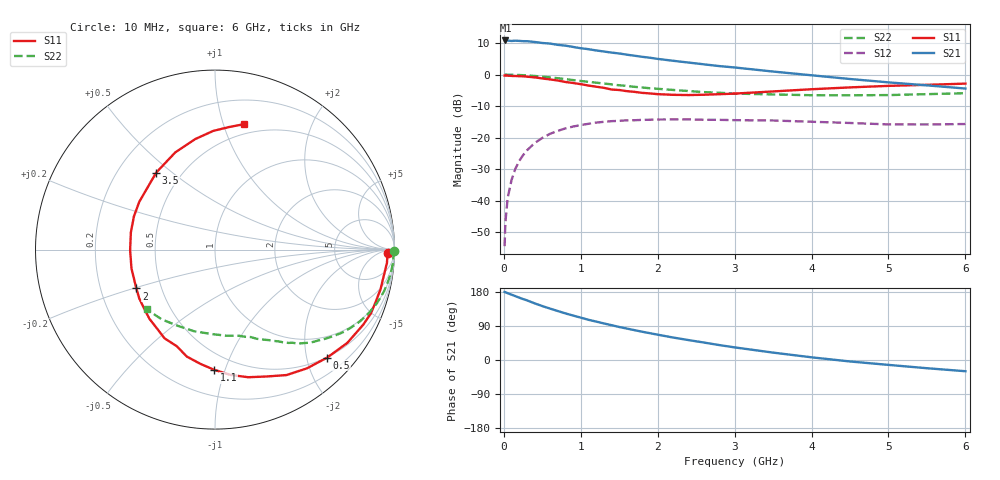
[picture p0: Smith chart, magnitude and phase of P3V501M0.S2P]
! SIEMENS Small Signal Semiconductors
! BFP181
! Si NPN RF Bipolar Junction Transistor in SOT143
! VCE = 0.5 V  IC = 1 mA
! Common Emitter S-Parameters:  March  1996
# GHz  S  MA  R  50
!  f  S11  S21  S12  S22
! GHz  MAG  ANG  MAG  ANG  MAG  ANG  MAG  ANG
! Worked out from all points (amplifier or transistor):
!   36 points, 10 MHz to 6 GHz, reference 50 ohm
!   highest |S21| = 10.8 dB at 20 MHz (marker M1)
!   |S21| within 3 dB of that: start of sweep to 1.158 GHz
!   unconditionally stable (mu >= 1): 2.652 GHz to end of sweep
!   at 250 MHz: K = 0.10, MSG = 18.1 dB, |S12| = -25.6 dB
!   at 1.4 GHz: K = 0.57, MSG = 10.9 dB, |S12| = -14.8 dB
!   at 6 GHz: K = 1.53, MAG = 1.3 dB, |S12| = -15.7 dB
!   S11 on the Smith chart (normalised r, x): 10 MHz: 42, -21; 500 MHz: 0.49, -2.39; 1.1 GHz: 0.38, -0.92; 2 GHz: 0.36, -0.20; 3.5 GHz: 0.36, +0.44; 6 GHz: 0.41, +1.18
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0.01  0.9622 -1.1  3.449 179.5  0.0019 87.5  0.9974 -0.4
0.02  0.9611 -1.7  3.473 179.1  0.0045 85.4  0.9982 -0.9
0.05  0.961 -4.4  3.458 176.2  0.0111 87.6  0.9952 -2.4
0.1  0.9513 -9.1  3.408 172.4  0.0212 84.2  0.9936 -4.7
0.15  0.9484 -13.5  3.445 168.5  0.0321 80.5  0.9891 -7.0
0.3  0.9256 -26.9  3.382 157.5  0.0627 72.1  0.9699 -13.9
0.4  0.902 -35.2  3.286 149.5  0.0819 66.4  0.9503 -18.3
0.5  0.8676 -43.9  3.167 142.3  0.0989 60.7  0.9273 -22.4
0.6  0.8369 -52.2  3.099 135.7  0.1148 55.7  0.9022 -26.2
0.8  0.7626 -68.0  2.875 123.0  0.1398 46.5  0.8485 -32.9
1.1  0.6698 -90.4  2.526 106.1  0.1656 34.6  0.7649 -41.5
1.3  0.6162 -104.8  2.321 96.5  0.178 27.7  0.721 -46.2
1.5  0.5685 -119.7  2.159 87.1  0.1845 22.2  0.6757 -50.2
1.8  0.5124 -140.7  1.911 74.5  0.1912 15.5  0.6232 -55.2
2  0.4887 -153.7  1.772 66.8  0.1936 11.5  0.5947 -58.2
2.2  0.4772 -167.2  1.654 59.3  0.1944 7.5  0.57 -61.7
2.8  0.4881 157.8  1.363 39.4  0.1914 -1.0  0.5145 -70.8
3.5  0.54 127.3  1.116 19.5  0.1869 -7.8  0.4838 -82.6
4  0.5852 112.2  0.974 7.1  0.1785 -11.6  0.4703 -93.0
4.5  0.6258 100.1  0.85 -3.9  0.1707 -14.6  0.4696 -104.5
5.5  0.6875 83.4  0.674 -21.7  0.1616 -13.5  0.4891 -127.3
6  0.7184 76.8  0.6 -29.6  0.1643 -12.7  0.5059 -138.8
